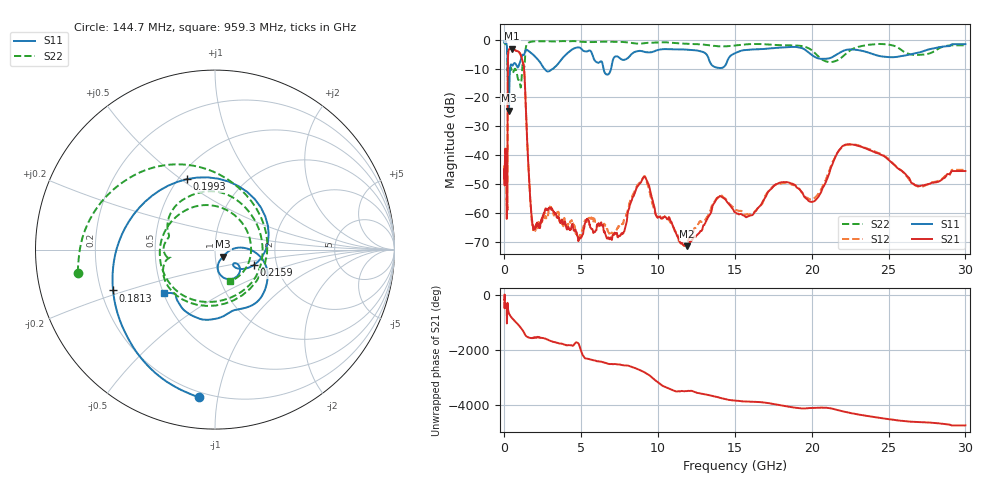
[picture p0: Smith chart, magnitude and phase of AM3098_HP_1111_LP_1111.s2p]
! Date/Time: Thu, Feb 28, 2019 8:48 AM
! Network Analyzer: Agilent Technologies E8364B Rev: A.07.50.67
! Sweep from 0.010 to 30.000 GHz, 1601 Points, Sweep Type: LOG
! Power Supply: 5.022 V, 0.002 A
# Hz S DB R 50
!freq MagS11 AngS11 MagS21 AngS21 MagS12 AngS12 MagS22 AngS22
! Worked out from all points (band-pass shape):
!   1601 points, 10 MHz to 30 GHz, reference 50 ohm
!   highest |S21| = -3.11 dB at 500.5 MHz (marker M1); lowest = -71.6 dB at 11.89 GHz (marker M2)
!   |S21| within 3 dB of the highest: 228.6 MHz to 1.112 GHz (883.5 MHz wide, 132 % of centre)
!   lowest |S11| = -24.5 dB at 293 MHz (marker M3), VSWR 1.13, Z = 54.5 - j4.29 ohm
!   |S11| at or under -10 dB: 210.2 MHz to 367.7 MHz (157.6 MHz wide, 54.5 % of centre); 2.603 GHz to 3.168 GHz (565.4 MHz wide, 19.6 % of centre); 6.447 GHz to 6.94 GHz (493.2 MHz wide, 7.37 % of centre)
!   |S22| runs from -16.6 to -0.4 dB; largest |S21 - S12| = 0.012
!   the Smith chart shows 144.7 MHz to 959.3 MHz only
!   S11 on the Smith chart (normalised r, x): 144.7 MHz: 0.17, -0.88; 181.3 MHz: 0.25, -0.18; 199.3 MHz: 0.55, +0.53; 215.9 MHz: 1.52, -0.28; 959.3 MHz: 0.50, -0.28
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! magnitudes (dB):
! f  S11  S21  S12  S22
! 10 MHz  -0.4  -45.3  -43.8  -0.6
! 38.04 MHz  -0.2  -41.4  -40.9  -0.8
! 96 MHz  -0.8  -39.3  -39.4  -1.5
! 144.7 MHz  -1.6  -57.2  -55.6  -2.2
! 181.3 MHz  -4.3  -58.7  -58.1  -5.4
! 199.3 MHz  -7.5  -34.8  -34.7  -10.7
! 215.9 MHz  -12.7  -11.1  -11.1  -9.7
! 293 MHz  -24.5  -3.3  -3.3  -11.4
! 356.2 MHz  -10.7  -3.2  -3.2  -10.2
! 500.5 MHz  -8.9  -3.1  -3.1  -11.3
! 550.5 MHz  -8.8  -3.3  -3.2  -11.4
! 959.3 MHz  -8.5  -4.3  -4.3  -14.2
! 1.27 GHz  -5.3  -9.7  -9.7  -9.9
! 1.731 GHz  -4.6  -58.8  -59.0  -0.7
! 2.084 GHz  -6.3  -64.1  -64.8  -0.5
! 7.926 GHz  -6.7  -63.8  -60.7  -0.9
! 9.072 GHz  -4.1  -47.6  -47.5  -1.2
! 11.89 GHz  -3.5  -71.6  -69.9  -1.4
! 14.02 GHz  -9.8  -54.2  -54.0  -2.3
! 20.1 GHz  -5.6  -56.1  -55.2  -4.1
! 22.56 GHz  -3.4  -36.3  -36.3  -3.5
! 30 GHz  -1.5  -45.5  -45.1  -1.9
